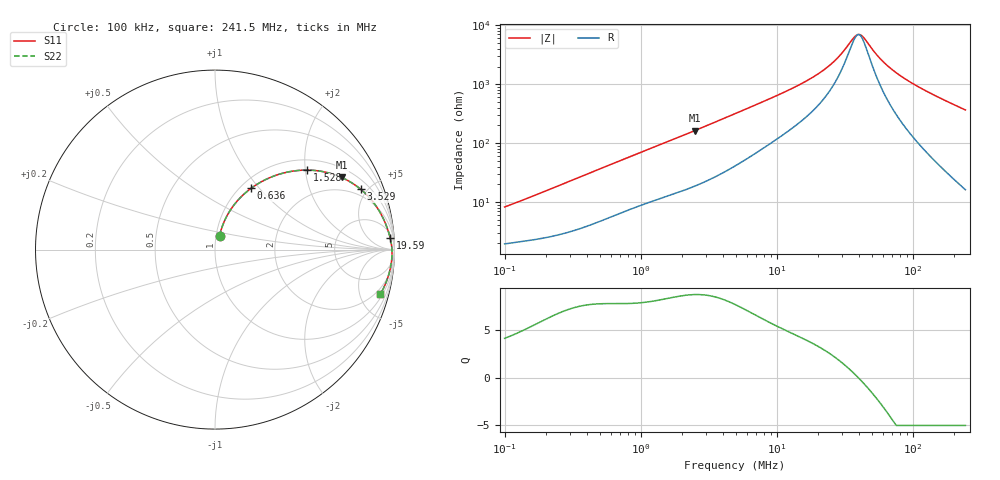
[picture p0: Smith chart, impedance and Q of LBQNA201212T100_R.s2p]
! LBQNA201212T100_R  S-PARAMETER MODEL  ( General Type )
! Model Generated by TAIYO YUDEN Corporation (http://www.ty-top.com)
! Version 1.0
! TAIYO YUDEN Control No. 191025NI43SB-FBB
! Copyright(c) 2019 TAIYO YUDEN CO.,LTD. All Rights Reserved.
! Product Description (link to TY-COMPAS)
! https://ds.yuden.co.jp/TYCOMPAS/or/detail?pn=LBQNA201212T100KR&u=M
! Products Name : Inductors
! Characteristics :
!  Inductance : 10 uH , SRF(min) : 32 MHz , DC Resistance(max) : 0.65 Ohm
!  Rated Current : Saturation :200 mA , Temp Rise : 300 mA (20 degC)
!  Case Size : 2.0 x 1.25 / 0.079 x 0.049 [mm/inch] , Thickness : 1.25 / 0.049 [mm/inch]
!  (Conditions: Temperature = 25 degC , DC Bias Current/Voltage = 0A / 0V)
! External Node Assignments :
!  1  o---GGG---o  2
! GND o---------o GND
! Frequency Range : 0.1MHz  -  241.513628MHz  [ 402 STEP ]
# MHz S RI R 50
! Freq[MHz].  S11 Real  S11 Imag  S21 Real  S21 Imag  S12 Real  S12 Imag  S22 Real  S22 Imag
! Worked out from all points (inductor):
!   401 points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, 100 kHz to 241.5 MHz, reference 50 ohm
!   read as one part in series: L = 12.4 uH near 104 kHz
!   highest Q = 8.7 at 2.486 MHz (marker M1), where L = 10.4 uH
!   self-resonance near 39.51 MHz
!   S11 on the Smith chart (normalised r, x): 100 kHz: 1.04, +0.16; 636 kHz: 1.12, +0.91; 1.528 MHz: 1.25, +2.04; 3.529 MHz: 1.54, +4.54; 19.59 MHz: 9, +28; 241.5 MHz: 1.32, -7.31
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0.1  0.0251 0.0766  0.9749 -0.0766  0.9749 -0.0766  0.0251 0.0766
0.193888  0.0437 0.1376  0.9563 -0.1376  0.9563 -0.1376  0.0437 0.1376
0.368674  0.0972 0.2371  0.9028 -0.2371  0.9028 -0.2371  0.0972 0.2371
0.635988  0.2022 0.3423  0.7978 -0.3423  0.7978 -0.3423  0.2022 0.3423
1.359207  0.4635 0.4409  0.5365 -0.4409  0.5365 -0.4409  0.4635 0.4409
1.52767  0.5118 0.443  0.4882 -0.443  0.4882 -0.443  0.5118 0.443
2.485784  0.7052 0.4021  0.2948 -0.4021  0.2948 -0.4021  0.7052 0.4021
3.529359  0.8124 0.3357  0.1876 -0.3357  0.1876 -0.3357  0.8124 0.3357
4.914404  0.8806 0.2655  0.1194 -0.2655  0.1194 -0.2655  0.8806 0.2655
10.91999  0.9562 0.1293  0.0438 -0.1293  0.0438 -0.1293  0.9562 0.1293
18.11814  0.9746 0.0711  0.0254 -0.0711  0.0254 -0.0711  0.9746 0.0711
19.58587  0.9766 0.0634  0.0234 -0.0634  0.0234 -0.0634  0.9766 0.0634
26.74611  0.9823 0.0343  0.0177 -0.0343  0.0177 -0.0343  0.9823 0.0343
30.65223  0.984 0.0222  0.016 -0.0222  0.016 -0.0222  0.984 0.0222
36.524  0.9855 0.00688  0.0145 -0.00688  0.0145 -0.00688  0.9855 0.00688
39.48278  0.9859 6.56e-05  0.0141 -6.56e-05  0.0141 -6.56e-05  0.9859 6.56e-05
42.68125  0.9862 -0.00679  0.0138 0.00679  0.0138 0.00679  0.9862 -0.00679
54.97721  0.9862 -0.0298  0.0138 0.0298  0.0138 0.0298  0.9862 -0.0298
66.79689  0.9851 -0.0488  0.0149 0.0488  0.0149 0.0488  0.9851 -0.0488
84.38097  0.9823 -0.074  0.0177 0.074  0.0177 0.074  0.9823 -0.074
110.8275  0.9761 -0.1082  0.0239 0.1082  0.0239 0.1082  0.9761 -0.1082
241.5136  0.921 -0.2485  0.079 0.2485  0.079 0.2485  0.921 -0.2485
